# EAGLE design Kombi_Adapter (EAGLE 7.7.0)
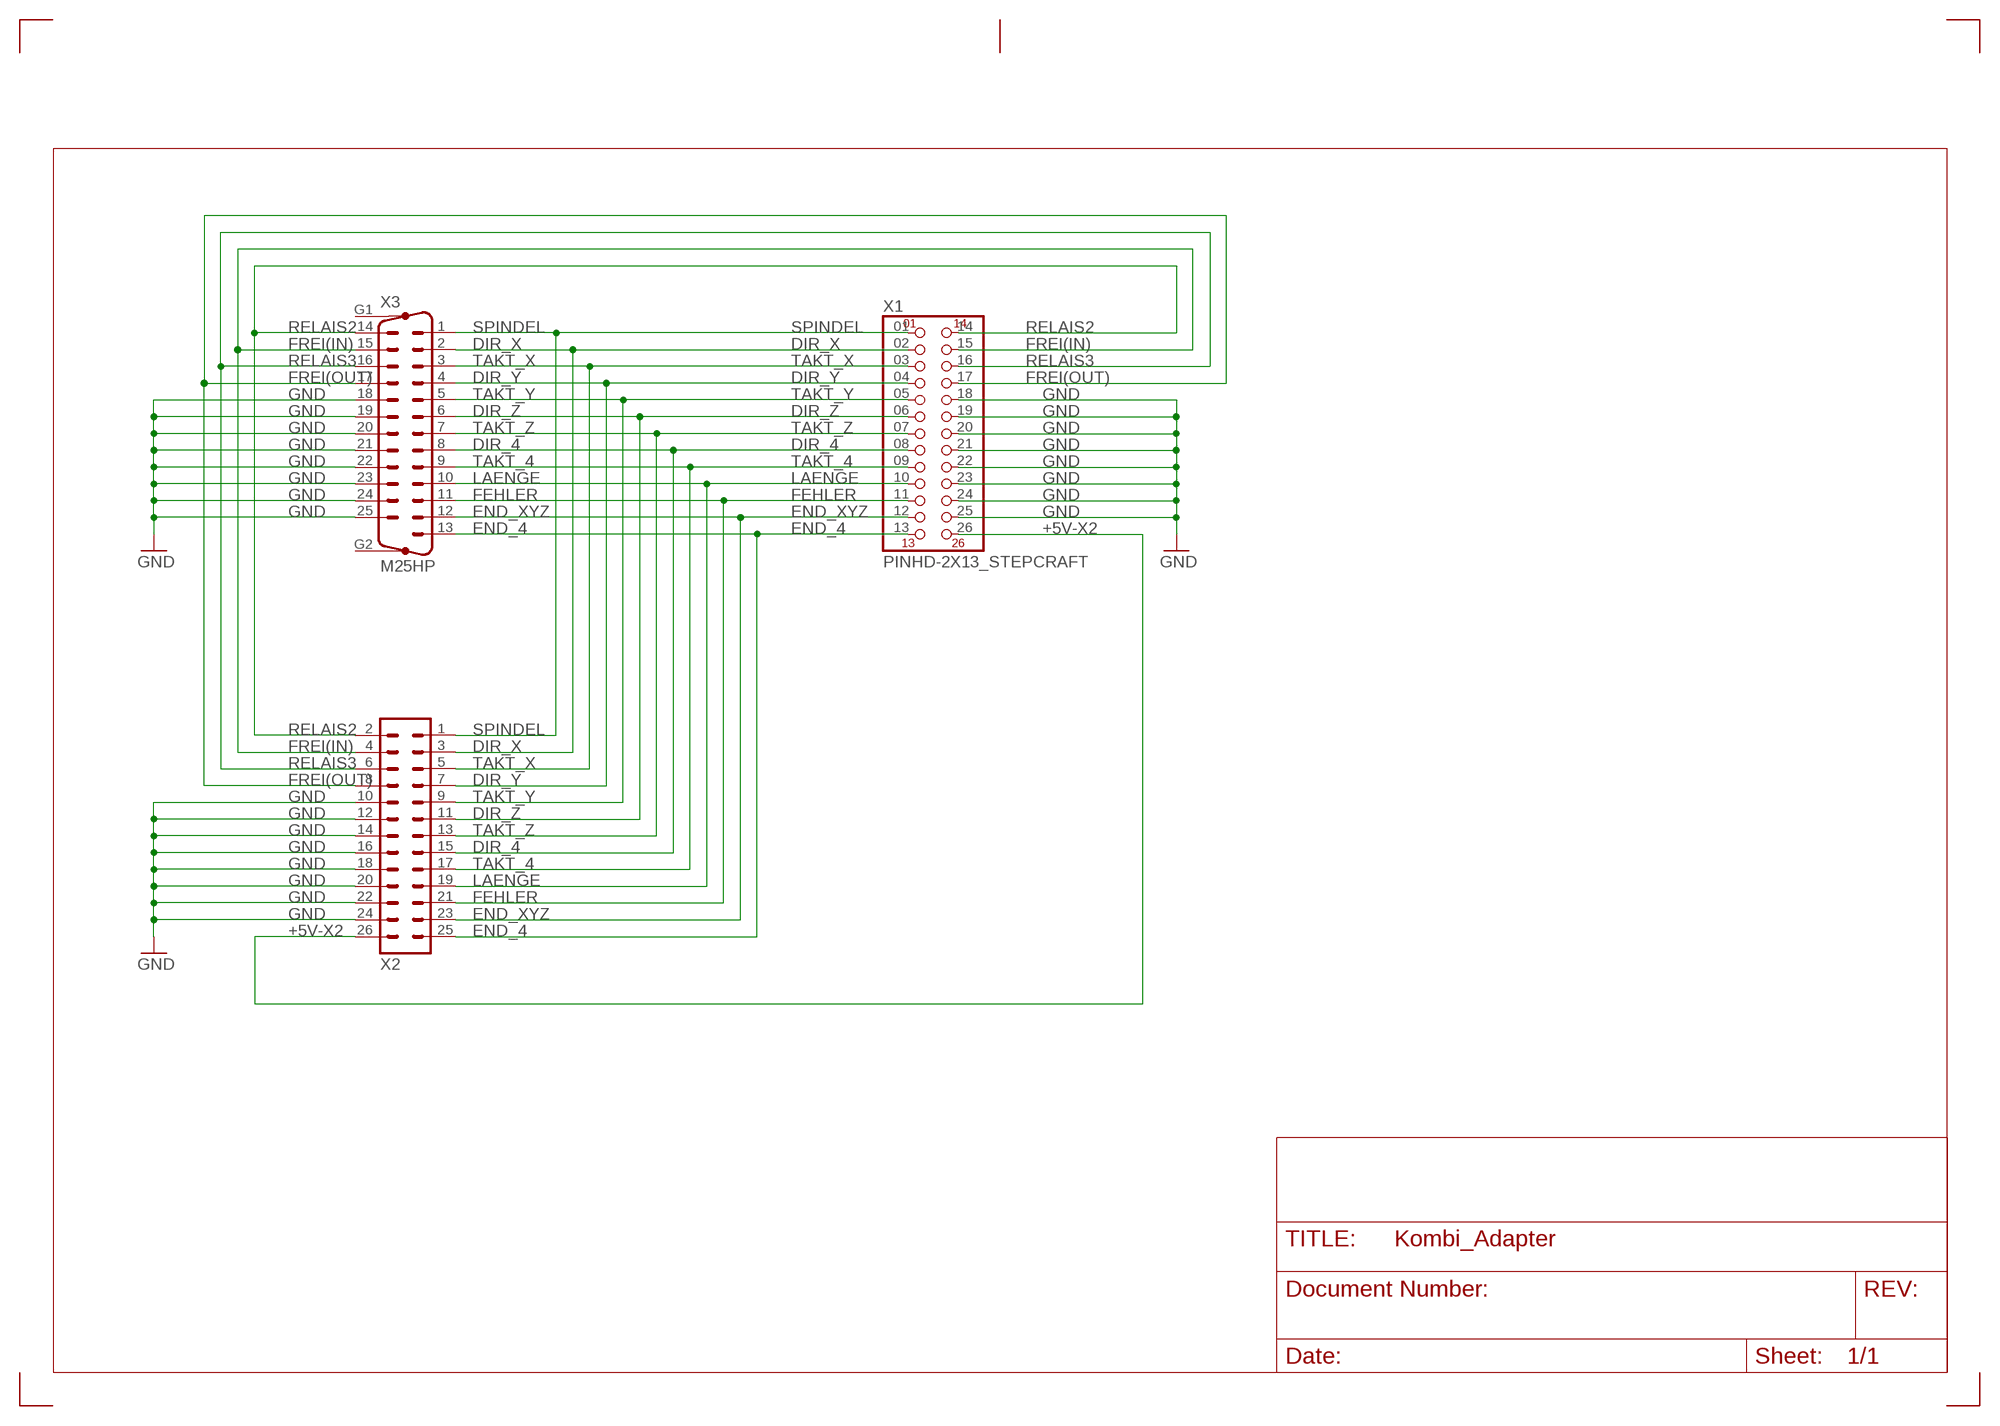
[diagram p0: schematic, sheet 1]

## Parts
X1  PINHD-2X13_STEPCRAFT  [2X13_90_STEPCRAFT]
X2  ML26  [ML26]
X3  M25HP  [M25HP]

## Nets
+5V-X2: X1.26 X2.26
DIR_4: X1.08 X2.15 X3.8
DIR_X: X1.02 X2.3 X3.2
DIR_Y: X1.04 X2.7 X3.4
DIR_Z: X1.06 X2.11 X3.6
END_4: X1.13 X2.25 X3.13
END_XYZ: X1.12 X2.23 X3.12
FEHLER: X1.11 X2.21 X3.11
FREI(IN): X1.15 X2.4 X3.15
FREI(OUT): X1.17 X2.8 X3.17
GND: X1.18 X1.19 X1.20 X1.21 X1.22 X1.23 X1.24 X1.25 X2.10 X2.12 X2.14 X2.16 X2.18 X2.20 X2.22 X2.24 X3.18 X3.19 X3.20 X3.21 X3.22 X3.23 X3.24 X3.25
LAENGE: X1.10 X2.19 X3.10
RELAIS2: X1.14 X2.2 X3.14
RELAIS3: X1.16 X2.6 X3.16
SPINDEL: X1.01 X2.1 X3.1
TAKT_4: X1.09 X2.17 X3.9
TAKT_X: X1.03 X2.5 X3.3
TAKT_Y: X1.05 X2.9 X3.5
TAKT_Z: X1.07 X2.13 X3.7
Unconnected: X3.G1 X3.G2

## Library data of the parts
X1 = con-pinhead:PINHD-2X13_STEPCRAFT
X2 = con-ml:ML26: HARTING; OC_FARNELL: unknown; OC_NEWARK: unknown
X3 = con-subd:M25?P

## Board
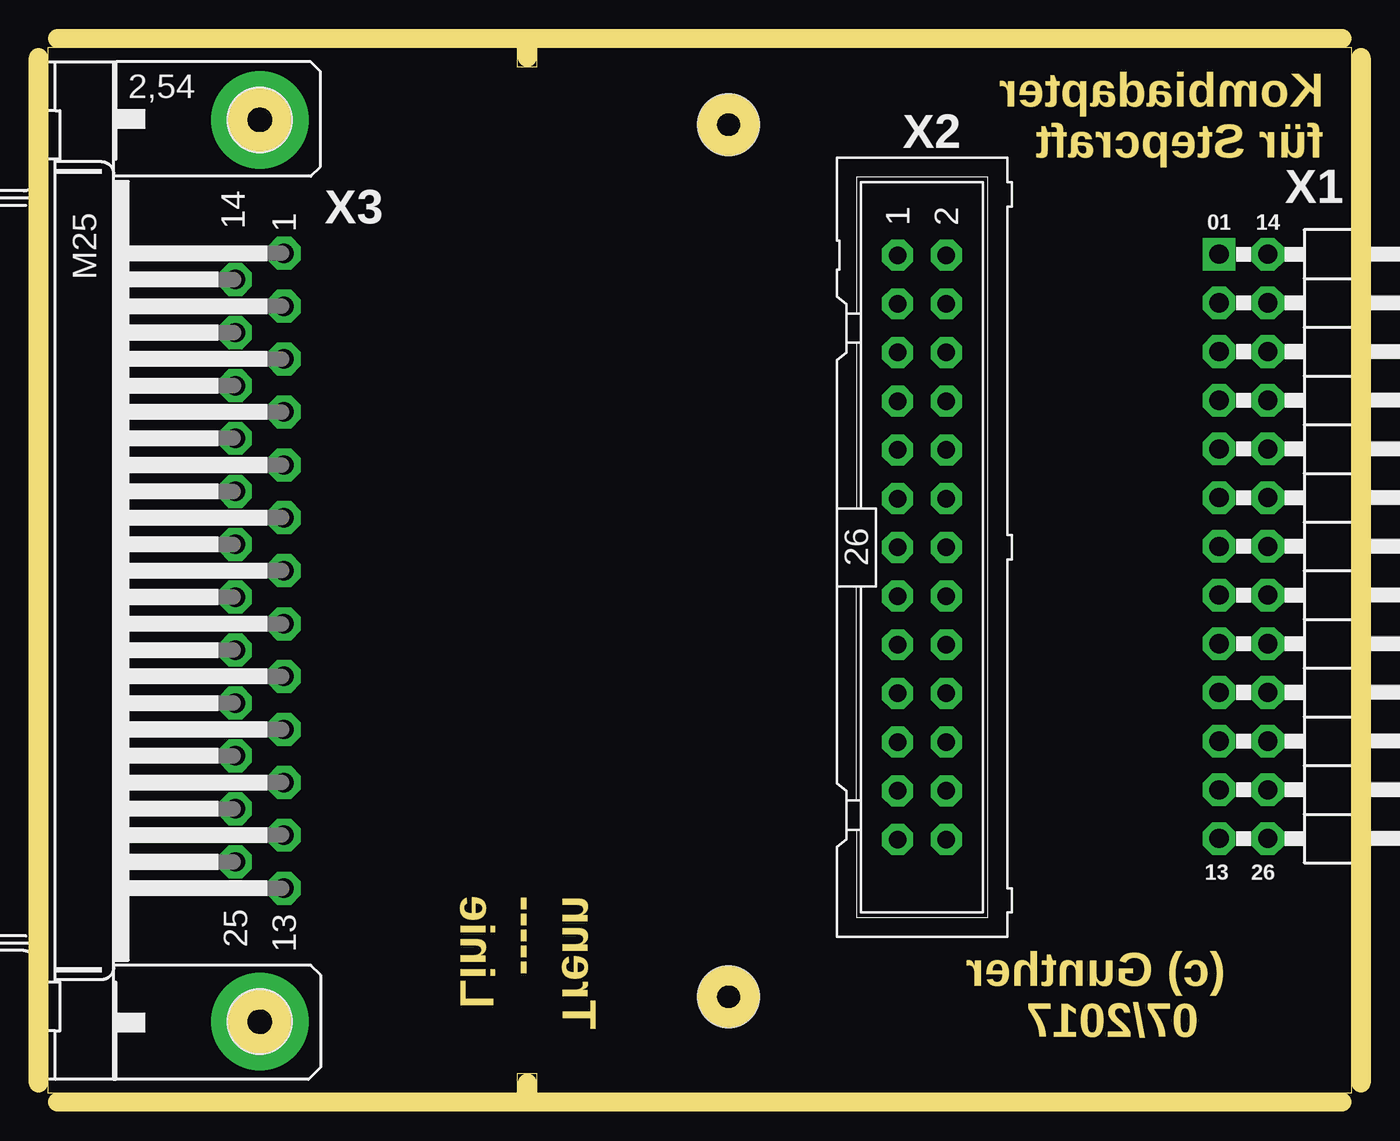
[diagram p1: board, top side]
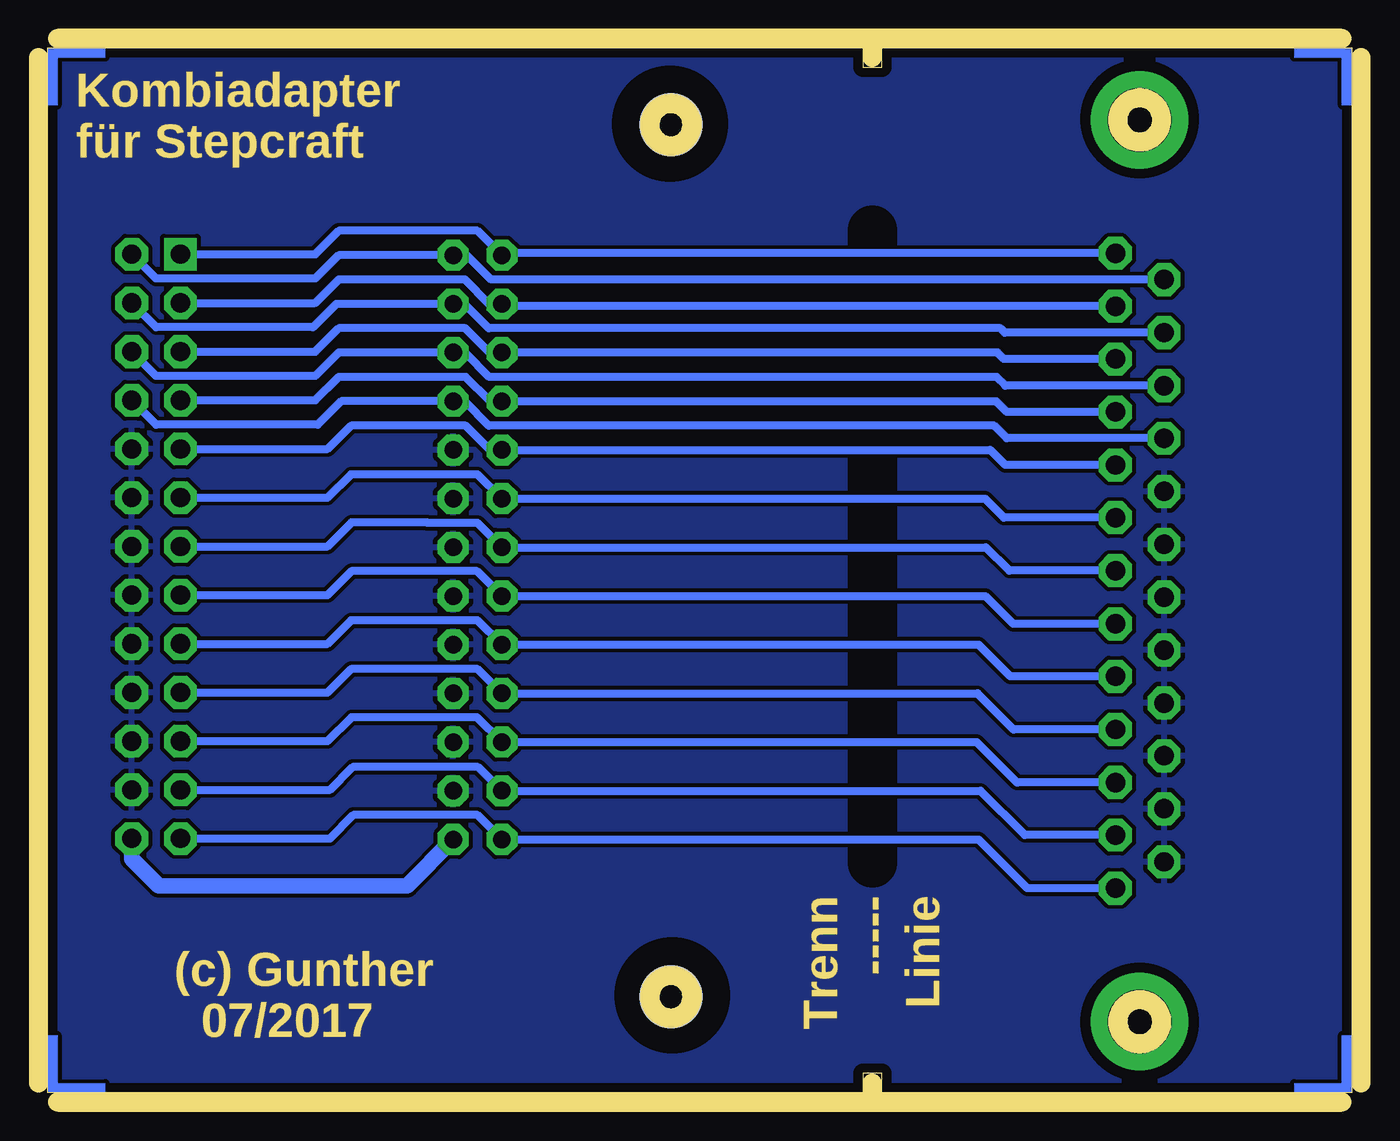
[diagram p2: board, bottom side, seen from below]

Size 68 x 54.5 mm. Coordinates in mm from the lower left corner, seen from the top.
Outline: 0,0 24.5,0 24.5,1 25.5,1 25.5,0 68,0 68,54.5 25.5,54.5 25.5,53.5 24.5,53.5 24.5,54.5 0,54.5 0,0
Copper layers (1*16): Top 0.035mm / dielectric 1.5mm / Bottom 0.035mm
Design rules "LP_fraesen *": minimum track width 10mil, minimum drill 24mil, track to track 8mil, track to pad 8mil, pad to pad 8mil, via to via 8mil, smd to smd 0mil, copper to edge 20mil, drill to drill 8mil, minimum pad ring 0.35mm, minimum via ring 15mil, stop-mask expansion 4mil, vias tented up to drill 0mil, thermal gap 10mil
Holes 3.2 mm at 35.5,50.5 35.5,5
bRestrict: area 32.9,47.9 to 38.2,53.2; area 32.8,2.4 to 38.1,7.7; area 8.3,48 to 13.8,53.6; area 8.3,0.9 to 13.8,6.5; 1 lines
Milling: 88 lines

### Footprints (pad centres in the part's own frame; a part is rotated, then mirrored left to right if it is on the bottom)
2X13_90_STEPCRAFT = drill 1 square: 01 -15.24,-1.27 | drill 1 octagon: 02 -12.7,-1.27; 03 -10.16,-1.27; 04 -7.62,-1.27; 05 -5.08,-1.27; 06 -2.54,-1.27; 07 0,-1.27; 08 2.54,-1.27; 09 5.08,-1.27; 10 7.62,-1.27; 11 10.16,-1.27; 12 12.7,-1.27; 13 15.24,-1.27; 14 -15.24,1.27; 15 -12.7,1.27; 16 -10.16,1.27; 17 -7.62,1.27; 18 -5.08,1.27; 19 -2.54,1.27; 20 0,1.27; 21 2.54,1.27; 22 5.08,1.27; 23 7.62,1.27; 24 10.16,1.27; 25 12.7,1.27; 26 15.24,1.27
ML26 = drill 0.914 octagon: 1 -15.24,-1.27; 2 -15.24,1.27; 3 -12.7,-1.27; 4 -12.7,1.27; 5 -10.16,-1.27; 6 -10.16,1.27; 7 -7.62,-1.27; 8 -7.62,1.27; 9 -5.08,-1.27; 10 -5.08,1.27; 11 -2.54,-1.27; 12 -2.54,1.27; 13 0,-1.27; 14 0,1.27; 15 2.54,-1.27; 16 2.54,1.27; 17 5.08,-1.27; 18 5.08,1.27; 19 7.62,-1.27; 20 7.62,1.27; 21 10.16,-1.27; 22 10.16,1.27; 23 12.7,-1.27; 24 12.7,1.27; 25 15.24,-1.27; 26 15.24,1.27
M25HP = drill 1.016 octagon: 1 -16.561,1.27; 2 -13.792,1.27; 3 -11.049,1.27; 4 -8.28,1.27; 5 -5.512,1.27; 6 -2.769,1.27; 7 0,1.27; 8 2.769,1.27; 9 5.512,1.27; 10 8.28,1.27; 11 11.049,1.27; 12 13.792,1.27; 13 16.561,1.27; 14 -15.189,-1.27; 15 -12.421,-1.27; 16 -9.652,-1.27; 17 -6.909,-1.27; 18 -4.14,-1.27; 19 -1.372,-1.27; 20 1.372,-1.27; 21 4.14,-1.27; 22 6.909,-1.27; 23 9.652,-1.27; 24 12.421,-1.27; 25 15.189,-1.27 | drill 3.302 pad 5.08: G1 -23.52,0; G2 23.52,0

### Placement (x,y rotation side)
X1  62.36,28.5 270 top
X2  45.59,28.45 270 top
X3  11.05,27.23 270 top

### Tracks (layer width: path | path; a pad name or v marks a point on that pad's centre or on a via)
+5V-X2
  Bottom 0.813: X1.26 63.63,12.19 62.23,10.79 49.28,10.79 X2.26
DIR_4
  Bottom 0.406: X3.8 17.65,24.46 19.1,25.91 X2.15 45.62,27.2 52.17,27.2 53.42,25.96 X1.08
DIR_X
  Bottom 0.406: X3.2 44.2,41.02 X2.3 44.98,41.15 46.25,42.42 52.83,42.42 54.05,41.2 X1.02
DIR_Y
  Bottom 0.406: X3.4 17.98,35.51 18.54,36.07 X2.7 44.93,36.07 46.2,37.34 52.83,37.34 54.05,36.12 X1.04
DIR_Z
  Bottom 0.406: X3.6 18.14,30 19.13,30.99 X2.11 45.59,32.26 52.2,32.26 53.42,31.04 X1.06
END_4
  Bottom 0.406: X3.13 16.92,10.67 19.46,13.21 X2.25 45.59,14.48 52.07,14.48 53.29,13.26 X1.13
END_XYZ
  Bottom 0.406: X3.12 17.04,13.44 19.36,15.75 X2.23 45.57,16.99 52.09,16.99 53.29,15.8 X1.12
FEHLER
  Bottom 0.406: X3.11 17.45,16.18 19.56,18.29 X2.21 45.62,19.58 52.17,19.58 53.42,18.34 X1.11
FREI(IN)
  Bottom 0.406: X1.15 62.36,39.93 54.18,39.93 52.96,41.15 X2.4 46.28,41.15 45.01,39.88 18.31,39.88 18.09,39.65 X3.15
FREI(OUT)
  Bottom 0.406: X1.17 62.36,34.85 53.92,34.85 52.7,36.07 X2.8 46.28,36.07 45.01,34.8 18.64,34.8 17.98,34.14 X3.17
GND
  pour Bottom (isolate 0.203, rank 3): 0,0 68.01,0 68.01,54.48 0,54.48
LAENGE
  Bottom 0.406: X3.10 17.63,18.95 19.51,20.83 X2.19 45.59,22.1 52.2,22.1 53.42,20.88 X1.10
RELAIS2
  Bottom 0.406: X1.14 62.36,42.47 54.05,42.47 52.83,43.69 X2.2 46.15,43.69 44.88,42.42 X3.14
RELAIS3
  Bottom 0.406: X1.16 62.36,37.39 54.05,37.39 52.83,38.61 X2.6 46.25,38.61 44.98,37.34 18.52,37.34 18.06,36.88 X3.16
SPINDEL
  Bottom 0.406: X3.1 44.22,43.79 X2.1 45.59,44.96 52.83,44.96 54.05,43.74 X1.01
TAKT_4
  Bottom 0.406: X3.9 17.8,21.72 19.46,23.37 X2.17 45.59,24.64 52.2,24.64 53.42,23.42 X1.09
TAKT_X
  Bottom 0.406: X3.3 18.14,38.28 18.47,38.61 X2.5 44.96,38.61 46.23,39.88 52.83,39.88 54.05,38.66 X1.03
TAKT_Y
  Bottom 0.406: X3.5 18.06,32.74 18.85,33.53 X2.9 44.93,33.53 46.2,34.8 52.2,34.8 53.42,33.58 X1.05
TAKT_Z
  Bottom 0.406: X3.7 17.86,27.23 19.07,28.45 X2.13 45.59,29.72 48.21,29.72 48.23,29.74 52.17,29.74 53.42,28.5 X1.07
(copper drawn outside any net)
  shapes: Bottom area x8

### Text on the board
Milling: Kombiadapter / für Stepcraft | Trenn / ----- / Linie | (c) Gunther / 07/2017
Document: Board 68,0 x 54,5 mm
